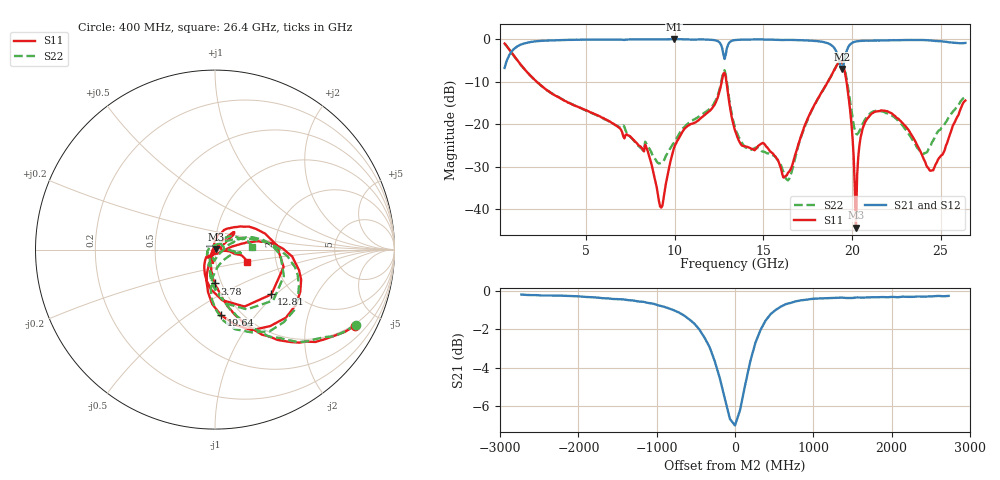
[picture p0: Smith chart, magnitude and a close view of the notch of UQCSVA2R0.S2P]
!  Part Number  UQCSVA2R0  Mounting Orientation: Horizontal
!  Description: Ultra Low ESR Microwave capacitors
!  Application: Coupling, Bypass, Tuning, DC Block
!  Filters, Matching
# GHZ S DB R 50
! Freq  |S11|  S11 Ph  |S21|  S21 Ph  |S12|  S12 Ph  |S22|  S22 Ph
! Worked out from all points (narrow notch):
!   401 points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, 400 MHz to 26.4 GHz, reference 50 ohm
!   highest |S21| = 0.01 dB at 9.955 GHz (marker M1); lowest = -7.0 dB at 19.45 GHz (marker M2)
!   notch at M2: 6.8 dB deep, 463 MHz wide at half that depth
!   lowest |S11| = -44.4 dB at 20.23 GHz (marker M3), VSWR 1.01, Z = 50.5 + j0.328 ohm
!   |S11| at or under -10 dB: 2.205 GHz to 12.65 GHz (10.45 GHz wide, 141 % of centre); 12.91 GHz to 18.64 GHz (5.73 GHz wide, 36.3 % of centre); 19.69 GHz to end of sweep
!   |S22| runs from -33.2 to -1.0 dB; largest |S21 - S12| = 0.01
!   S11 on the Smith chart (normalised r, x): 400 MHz: 0.93, -3.71; 3.78 GHz: 0.93, -0.36; 12.81 GHz: 1.58, -0.94; 19.64 GHz: 0.81, -0.68; 26.4 GHz: 1.41, -0.20
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0.4  -1.04 -28.6  -6.79 61.2  -6.80 61.1  -1.02 -28.1
1.57  -7.32 -69.2  -0.95 20.6  -0.96 20.5  -7.33 -68.0
3.78  -14.50 -90.5  -0.20 -2.5  -0.21 -2.6  -14.46 -92.1
4.755  -16.29 -95.1  -0.14 -8.3  -0.15 -8.4  -16.37 -98.5
8.46  -26.15 -123.7  -0.06 -26.5  -0.06 -26.6  -24.99 -90.3
9.11  -38.13 179.9  -0.08 -29.2  -0.08 -29.3  -29.27 -45.6
9.305  -39.19 123.1  -0.08 -29.9  -0.08 -30.1  -28.99 -25.3
9.955  -25.65 89.1  0.01 -33.3  0.01 -33.4  -24.37 10.9
12.425  -13.76 38.5  -0.49 -51.9  -0.49 -51.9  -13.21 18.5
12.815  -7.93 -38.4  -4.67 -43.9  -4.57 -44.3  -7.31 -41.2
13.4  -21.47 -131.4  -0.22 -41.4  -0.24 -41.4  -20.79 -107.0
16.39  -31.43 -53.7  -0.18 -60.2  -0.19 -60.3  -33.23 112.1
17.755  -16.47 12.5  -0.39 -68.4  -0.38 -68.5  -16.55 23.8
18.86  -8.39 0.7  -1.49 -81.4  -1.49 -81.7  -8.40 -2.6
19.445  -5.59 -54.2  -7.01 -63.5  -6.90 -63.7  -5.23 -56.4
19.64  -8.73 -84.8  -3.68 -45.1  -3.66 -45.6  -8.02 -83.4
20.225  -44.36 32.4  -0.55 -60.9  -0.56 -61.2  -22.20 -58.8
20.745  -19.49 45.3  -0.37 -68.2  -0.40 -68.4  -18.85 -10.5
22.11  -17.22 39.6  -0.29 -78.1  -0.29 -78.2  -17.69 -6.0
23.93  -27.02 26.9  -0.22 -89.9  -0.20 -89.9  -26.66 26.3
24.515  -30.89 15.5  -0.36 -94.2  -0.36 -94.3  -24.26 56.6
26.4  -14.45 -21.4  -0.89 -104.5  -0.89 -104.6  -13.68 3.9
